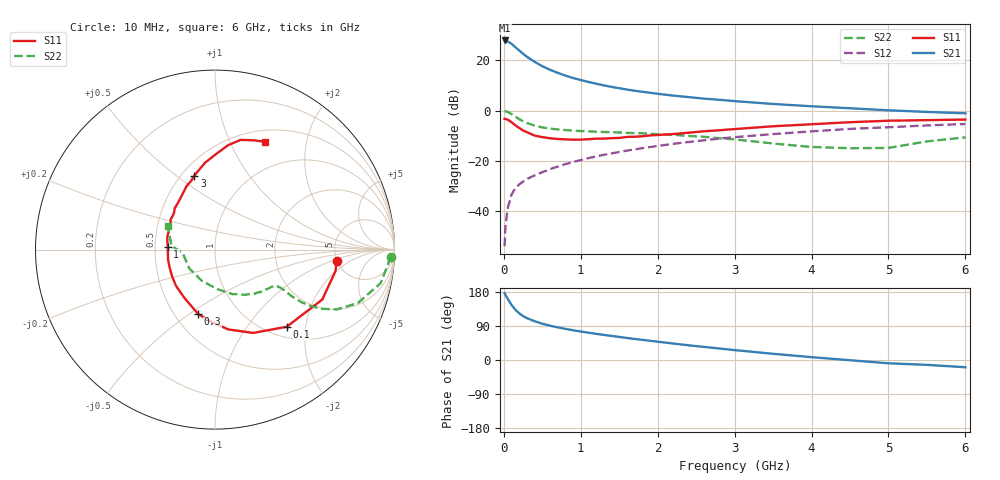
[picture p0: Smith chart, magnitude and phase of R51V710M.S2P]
! SIEMENS Small Signal Semiconductors
! BFR183
! Si NPN RF Bipolar Junction Transistor in SOT23
! VCE = 1.75 V  IC = 10 mA
! Common Emitter S-Parameters:  May  1996
# GHz  S  MA  R  50
!  f  S11  S21  S12  S22
! GHz  MAG  ANG  MAG  ANG  MAG  ANG  MAG  ANG
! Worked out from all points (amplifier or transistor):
!   36 points, 10 MHz to 6 GHz, reference 50 ohm
!   highest |S21| = 27.9 dB at 10 MHz (marker M1)
!   |S21| within 3 dB of that: start of sweep to 161.5 MHz
!   unconditionally stable (mu >= 1): 741 MHz to 2.516 GHz
!   at 250 MHz: K = 0.64, MSG = 25.4 dB, |S12| = -28.3 dB
!   at 1.4 GHz: K = 1.06, MAG = 11.7 dB, |S12| = -17.1 dB
!   at 6 GHz: K = 0.90, MSG = 2.1 dB, |S12| = -5.3 dB
!   S11 on the Smith chart (normalised r, x): 10 MHz: 5.00, -1.18; 100 MHz: 1.20, -1.58; 300 MHz: 0.65, -0.54; 1 GHz: 0.58, +0.02; 3 GHz: 0.58, +0.58; 6 GHz: 0.63, +1.36
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0.01  0.6817 -5.3  24.86 176.3  0.002 91.0  0.9788 -2.3
0.02  0.6818 -10.2  24.62 172.1  0.0048 82.2  0.9683 -4.7
0.05  0.6592 -25.0  23.85 161.4  0.0114 78.8  0.9415 -11.5
0.1  0.5868 -47.1  21.35 145.5  0.0214 70.4  0.8497 -20.5
0.15  0.5107 -65.4  18.22 132.5  0.0286 65.5  0.7567 -26.1
0.2  0.4507 -80.6  15.69 123.2  0.0339 62.5  0.6758 -29.2
0.25  0.4015 -93.4  13.5 115.9  0.0386 61.6  0.6107 -30.7
0.3  0.3716 -104.5  11.77 110.4  0.0433 61.8  0.5648 -31.3
0.4  0.3181 -122.6  9.321 102.4  0.0513 62.0  0.503 -31.3
0.5  0.2962 -137.4  7.634 95.7  0.0594 63.1  0.4622 -30.7
0.6  0.2814 -148.5  6.489 90.5  0.0683 64.2  0.4375 -30.3
0.7  0.2717 -158.4  5.641 86.1  0.0766 64.7  0.4215 -30.2
0.8  0.2672 -168.0  4.964 82.1  0.0859 64.5  0.4093 -30.4
1  0.2639 176.7  4.046 75.2  0.1036 64.8  0.392 -31.1
1.1  0.2695 170.2  3.712 72.1  0.113 64.7  0.386 -32.2
1.6  0.2986 145.8  2.617 58.1  0.1596 62.0  0.3602 -38.0
2.2  0.3408 125.3  1.984 43.5  0.2172 57.0  0.3296 -48.3
3  0.4282 105.6  1.542 26.1  0.2953 48.1  0.2675 -68.2
3.5  0.4868 96.6  1.353 16.4  0.3406 41.8  0.2209 -86.6
4.5  0.5866 82.8  1.112 -0.6  0.4317 29.1  0.1778 -143.6
5.5  0.6454 70.7  0.94 -12.8  0.5062 17.1  0.2434 174.9
6  0.662 65.3  0.883 -19.1  0.5404 9.3  0.2929 153.8
